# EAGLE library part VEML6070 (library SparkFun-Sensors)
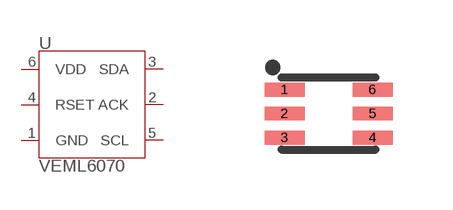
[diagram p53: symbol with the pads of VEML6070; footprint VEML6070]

Designator prefix U

## VEML6070" (PROD_ID: SEN-14367; VALUE: VEML6070)  [VEML6070]
1  GND
2  ACK
3  SDA
4  RSET
5  SCL
6  VDD

## Footprint VEML6070 (pad centres in mm)
VEML6070 - Package for the VEML6070 Specifications: Pin count: 6 Pin pitch: .6mm Area: 2.35mm x 1.8mm Datasheet referenced for footprint
smd 1 x 0.35: 1 -1.1,0.6; 2 -1.1,0; 3 -1.1,-0.6; 4 1.1,-0.6; 5 1.1,0; 6 1.1,0.6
